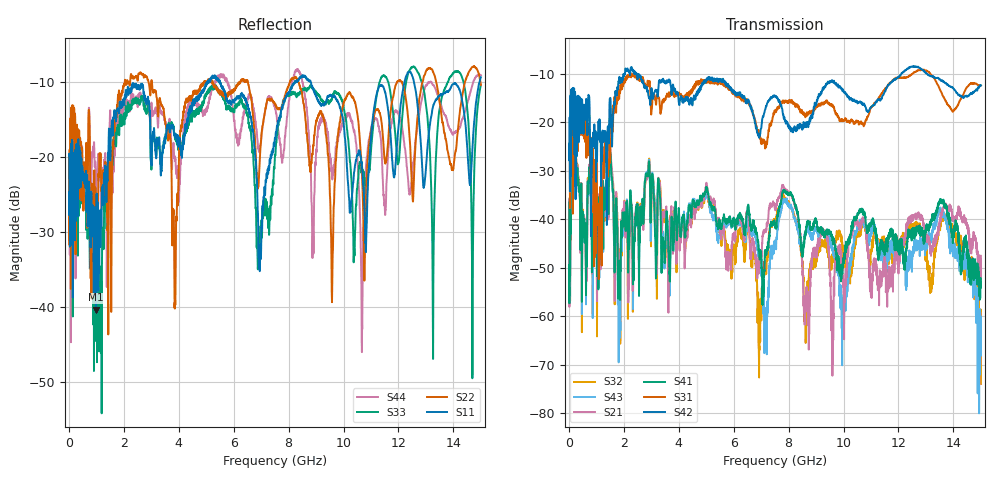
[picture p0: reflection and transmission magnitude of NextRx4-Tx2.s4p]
!  = SDD11
!  = SDD12
!  = SDC11
!  = SDC12
!  = SDD21
!  = SDD22
!  = SDC21
!  = SDC22
!  = SCD11
!  = SCD12
!  = SCC11
!  = SCC12
!  = SCD21
!  = SCD22
!  = SCC21
!  = SCC22
! FILE: N:\QM 2007\Prüfprotokolle\Highspeed\Konfektionierte Ltg\L45593-D106\D30\8216\0002\Next  Platine 2\NextRx4-Tx2.s4p
# MHz S DB R 50.00
! FREQ  S11  S12  S13  S14
!  S21  S22  S23  S24
!  S31  S32  S33  S34
!  S41  S42  S43  S44
!  DB  ANG  DB  ANG  DB  ANG  DB  ANG
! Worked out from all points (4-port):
!   2999 points, 10 MHz to 15 GHz, reference 50 ohm
!   strongest paths, dB at 10 MHz, 3.755 GHz, 7.505 GHz, 11.26 GHz, 15 GHz:
!     S42: -25.2, -13.1, -14.6, -15.4, -12.4
!     S31: -25.2, -13.8, -18.0, -15.2, -12.4
!     S41: -52.8, -40.4, -40.9, -47.9, -53.1
!     S21: -46.6, -40.8, -37.6, -52.3, -47.6
!     S43: -48.7, -41.3, -44.8, -45.4, -60.3
!     S32: -43.8, -41.2, -40.4, -44.9, -74.0
!   lowest |S11| = -40.4 dB at 990 MHz (marker M1), VSWR 1.02, Z = 49.5 - j0.835 ohm
!   |S11| at or under -10 dB: start of sweep to 5.044 GHz; 5.502 GHz to 8.223 GHz (2.721 GHz wide, 39.7 % of centre); 8.816 GHz to 12.21 GHz (3.399 GHz wide, 32.3 % of centre)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
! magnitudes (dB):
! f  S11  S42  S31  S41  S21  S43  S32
! 10 MHz  -19.7  -25.2  -25.2  -52.8  -46.6  -48.7  -43.8
! 990 MHz  -40.4  -32.3  -35.9  -39.7  -41.4  -42.0  -43.1
! 2.225 GHz  -10.9  -10.3  -10.6  -35.4  -38.2  -35.7  -38.0
! 7.175 GHz  -23.3  -16.7  -25.0  -46.4  -42.4  -66.1  -50.0
! 7.835 GHz  -12.5  -19.2  -16.0  -34.1  -33.7  -36.1  -35.6
! 13.69 GHz  -11.5  -11.9  -15.2  -36.9  -36.9  -39.9  -39.4
! 15 GHz  -9.3  -12.4  -12.4  -53.1  -47.6  -60.3  -74.0
